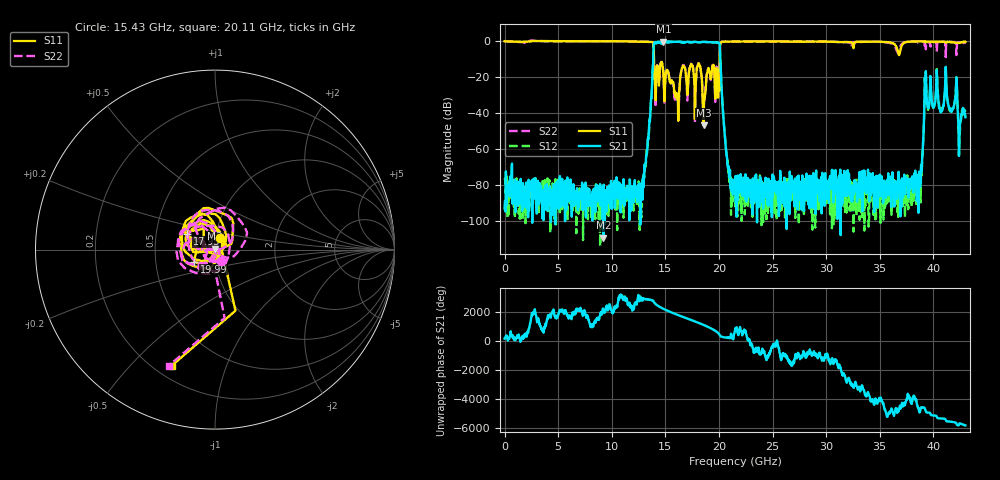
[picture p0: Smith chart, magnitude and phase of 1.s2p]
! 5/12/2023 2:31:54 PM
! D:\_XLC\ZBF13-C17-6G-753\1.S2P
! CHANNEL.1
! TR.MEASUREMENT
! CORRECTED.DATA
! RF.CORRECTION: FULL.TWO.PORT.CAL.PORT.1.2
! AVERAGING.OFF
! IF.BANDWIDTH: 10KHZ
! SWEEPTYPE:  FREQ.SWEEP(Linear)
! Reference Plane Port Info
! PORT:  PORT1  PORT2
! DISTANCE:  0  m  0  m
! TIME:  0  s  0  s
! PHASE.OFFSET:  0 °  0 °
! LOSS:  0  dB  0  dB
! REF.LOSS:  0  dB  0  dB
! REF.FREQ:  0  Hz  0  Hz
! Power Info
! POWER:  0  dBm  0  dBm
! EFF.POWER:  0  dBm  0  dBm
! SOURCE.ATTEN:  0  dB  0  dB
! TEST.ATTEN:  0  dB  0  dB
# GHZ S RI R 50.0
! FREQ.GHZ  S11RE  S11IM  S21RE  S21IM  S12RE  S12IM  S22RE  S22IM
!; PortSelection: Port_12
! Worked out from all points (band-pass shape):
!   1434 points, 10 MHz to 42.99 GHz, reference 50 ohm
!   highest |S21| = -0.32 dB at 14.83 GHz (marker M1); lowest = -109.4 dB at 9.218 GHz (marker M2)
!   |S21| within 3 dB of the highest: 13.91 GHz to 20.08 GHz (6.171 GHz wide, 36.3 % of centre)
!   lowest |S11| = -47.0 dB at 18.58 GHz (marker M3), VSWR 1.01, Z = 49.9 + j0.443 ohm
!   |S11| at or under -10 dB: 13.94 GHz to 20.07 GHz (6.138 GHz wide, 36.1 % of centre)
!   |S22| runs from -45.5 to 0.3 dB; largest |S21 - S12| = 0.16
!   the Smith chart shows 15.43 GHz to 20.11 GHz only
!   S11 on the Smith chart (normalised r, x): 15.43 GHz: 1.04, +0.14; 17.95 GHz: 0.72, +0.13; 19.99 GHz: 0.79, -0.11; 20.11 GHz: 0.27, -0.66
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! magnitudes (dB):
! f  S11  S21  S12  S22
! 10 MHz  -0.2  -93.2  -76.3  0.0
! 7.179 GHz  -0.2  -82.2  -91.5  -0.1
! 9.218 GHz  -0.2  -109.4  -95.6  -0.2
! 12.82 GHz  -0.4  -84.4  -92.0  -0.4
! 13.36 GHz  -0.5  -55.2  -58.1  -0.5
! 13.99 GHz  -21.2  -1.1  -0.9  -18.6
! 14.35 GHz  -18.6  -0.6  -0.8  -19.1
! 14.83 GHz  -18.7  -0.3  -0.6  -19.1
! 15.43 GHz  -22.8  -0.4  -0.7  -22.6
! 16.06 GHz  -30.4  -0.6  -0.5  -28.7
! 16.66 GHz  -13.8  -0.6  -0.6  -13.5
! 17.95 GHz  -15.1  -0.7  -0.6  -14.9
! 18.58 GHz  -47.0  -0.6  -0.5  -39.5
! 19.99 GHz  -17.4  -1.1  -1.2  -16.2
! 20.11 GHz  -3.2  -6.3  -6.3  -3.1
! 20.8 GHz  -0.4  -69.3  -68.4  -0.3
! 21.52 GHz  -0.4  -80.9  -82.8  -0.3
! 28.69 GHz  -0.4  -78.9  -89.9  -0.3
! 35.85 GHz  -0.8  -81.9  -89.3  -1.0
! 38.64 GHz  -0.3  -80.0  -85.9  -0.6
! 39.39 GHz  -0.3  -33.5  -33.8  -0.7
! 42.99 GHz  -0.6  -42.4  -42.4  -0.7
